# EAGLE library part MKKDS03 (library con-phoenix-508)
PHOENIX
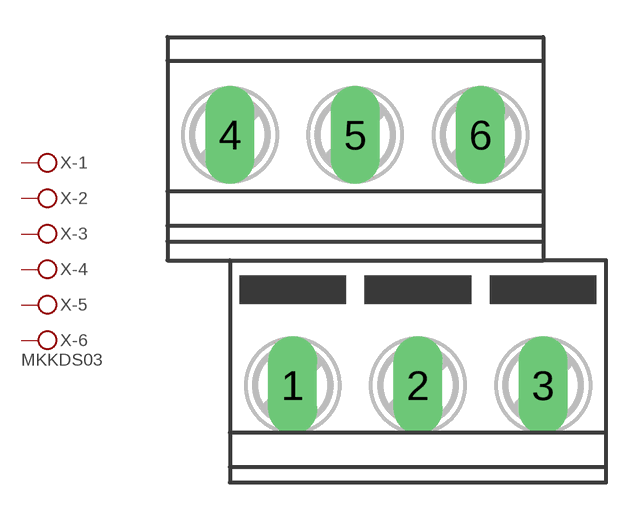
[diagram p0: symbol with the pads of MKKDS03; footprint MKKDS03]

Designator prefix X; gates -1=KL -2=KL -3=KL -4=KL -5=KL -6=KLV

## MKKDS03 (MF: FARNELL; MPN: 1721731; OC_FARNELL: 3041347; OC_NEWARK: 71C4104)  [MKKDS03]
1  -1:KL  pas
2  -2:KL  pas
3  -3:KL  pas
4  -4:KL  pas
5  -5:KL  pas
6  -6:KL  pas

## Footprint MKKDS03 (pad centres in mm)
PHOENIX MKKDSN 1,5/ 8-5,08 Source: http://eshop.phoenixcontact.com .. 1726202.pdf
drill 1.321 long: 1 -3.81,-5.08; 2 1.27,-5.08; 3 6.35,-5.08; 4 -6.35,5.08; 5 -1.27,5.08; 6 3.81,5.08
